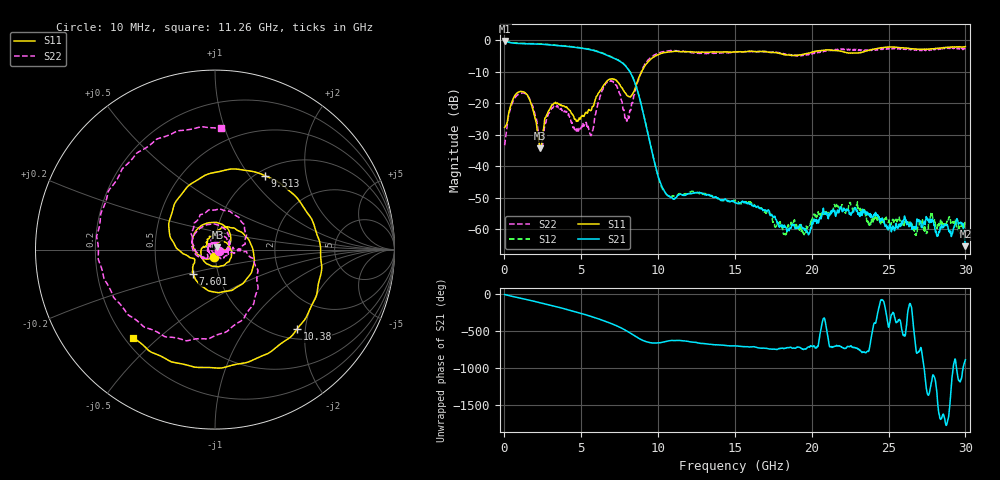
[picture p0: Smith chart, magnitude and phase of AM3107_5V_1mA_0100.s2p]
# Hz S DB R 50.0
!freq dBS11 angS11 dBS21 angS21 dBS12 angS12 dBS22 angS22
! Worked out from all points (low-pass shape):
!   1601 points, 10 MHz to 30 GHz, reference 50 ohm
!   highest |S21| = -0.20 dB at 10 MHz (marker M1); lowest = -65.5 dB at 30 GHz (marker M2)
!   |S21| within 3 dB of the highest: start of sweep to 5.79 GHz
!   lowest |S11| = -34.3 dB at 2.315 GHz (marker M3), VSWR 1.04, Z = 51.4 + j1.38 ohm
!   |S11| at or under -10 dB: start of sweep to 8.932 GHz
!   |S22| runs from -34.5 to -2.2 dB; largest |S21 - S12| = 0.02
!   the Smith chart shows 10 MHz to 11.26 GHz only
!   S11 on the Smith chart (normalised r, x): 10 MHz: 0.99, -0.08; 7.601 GHz: 0.76, -0.21; 9.513 GHz: 1.09, +1.20; 10.38 GHz: 1.20, -1.80; 11.26 GHz: 0.23, -0.42
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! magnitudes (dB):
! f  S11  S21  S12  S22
! 10 MHz  -27.7  -0.2  0.0  -33.4
! 516.1 MHz  -19.2  -0.8  -0.7  -19.8
! 1.228 GHz  -16.4  -1.1  -1.0  -16.7
! 1.828 GHz  -21.5  -1.1  -1.0  -20.8
! 2.315 GHz  -34.3  -1.2  -1.1  -34.2
! 3.309 GHz  -19.8  -1.6  -1.5  -20.8
! 5.015 GHz  -24.1  -2.5  -2.4  -27.7
! 5.671 GHz  -21.9  -3.1  -3.0  -29.7
! 6.72 GHz  -12.7  -4.8  -4.7  -13.0
! 7.601 GHz  -14.9  -6.9  -6.8  -19.0
! 7.995 GHz  -17.6  -8.8  -8.7  -25.1
! 9.513 GHz  -6.1  -33.6  -33.4  -5.5
! 10.02 GHz  -4.5  -43.6  -43.6  -4.1
! 10.38 GHz  -3.9  -47.6  -47.9  -3.6
! 11.26 GHz  -3.5  -49.5  -49.2  -3.4
! 15.01 GHz  -3.7  -51.6  -50.9  -3.7
! 18.25 GHz  -4.5  -59.1  -61.6  -4.4
! 20.01 GHz  -3.8  -57.8  -57.0  -4.3
! 21.98 GHz  -3.5  -54.5  -52.3  -3.0
! 25.01 GHz  -2.1  -59.5  -57.2  -2.7
! 29.55 GHz  -2.0  -58.5  -60.7  -2.5
! 30 GHz  -2.0  -65.5  -58.7  -2.4
